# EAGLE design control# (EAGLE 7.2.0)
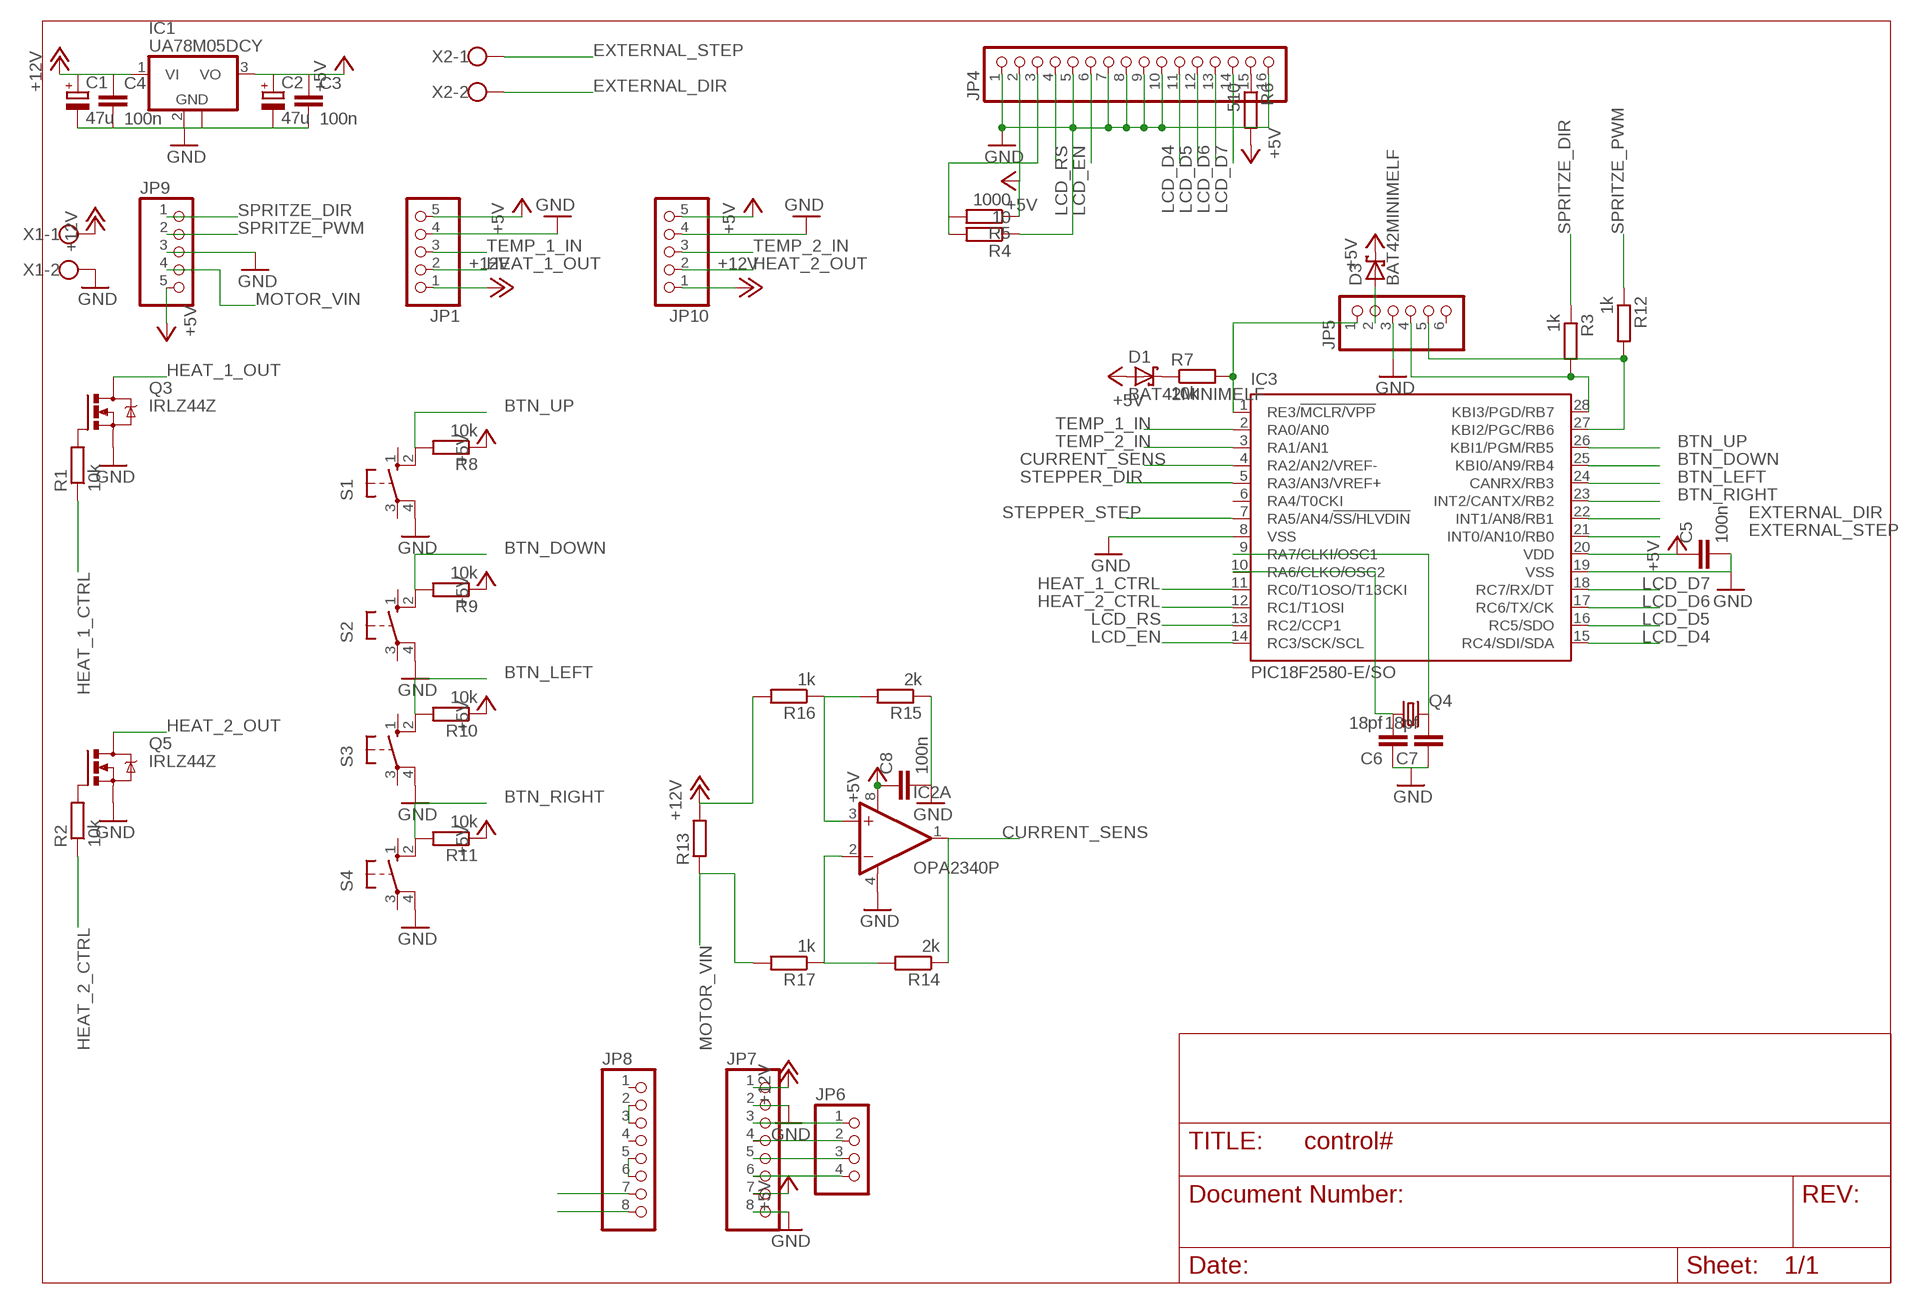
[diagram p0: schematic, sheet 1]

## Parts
C1  47u  CPOL-EU153CLV-0605  [153CLV-0605]
C2  47u  CPOL-EU153CLV-0605  [153CLV-0605]
C3  100n  C-EUC0603  [C0603]
C4  100n  C-EUC0603  [C0603]
C5  100n  C-EUC0603  [C0603]
C6  18pf  C-EUC0603  [C0603]
C7  18pf  C-EUC0603  [C0603]
C8  100n  C-EUC0603  [C0603]
D1  BAT42MINIMELF  [MINIMELF]
D3  BAT42MINIMELF  [MINIMELF]
IC1  UA78M05DCY  [SOT223]
IC2  OPA2340P  [DIL08]
IC3  PIC18F2580-E/SO  [SO28W]
JP1  PINHD-1X5_2.54  [1X05]
JP4  PINHD-1X16_2.54  [1X16]
JP5  PINHD-1X6_2.54  [1X06]
JP6  PINHD-1X4_2.54  [1X04]
JP7  PINHD-1X8_2.54  [1X08]
JP8  PINHD-1X8_2.54  [1X08]
JP9  PINHD-1X5_2.54  [1X05]
JP10  PINHD-1X5_2.54  [1X05]
Q3  IRLZ44Z  [TO220BH]
Q4  CRYSTALCTS406  [CTS406]
Q5  IRLZ44Z  [TO220BH]
R1  10k  R-EU_R0402  [R0402]
R2  10k  R-EU_R0402  [R0402]
R3  1k  R-EU_R0402  [R0402]
R4  10  R-EU_R0402  [R0402]
R5  1000  R-EU_R0402  [R0402]
R6  510  R-EU_R0402  [R0402]
R7  10k  R-EU_R0402  [R0402]
R8  10k  R-EU_R0402  [R0402]
R9  10k  R-EU_R0402  [R0402]
R10  10k  R-EU_R0402  [R0402]
R11  10k  R-EU_R0402  [R0402]
R12  1k  R-EU_R0402  [R0402]
R13  R-EU_R6332W  [R6332W]
R14  2k  R-EU_R0402  [R0402]
R15  2k  R-EU_R0402  [R0402]
R16  1k  R-EU_R0402  [R0402]
R17  1k  R-EU_R0402  [R0402]
S1  10-XX  [B3F-10XX]
S2  10-XX  [B3F-10XX]
S3  10-XX  [B3F-10XX]
S4  10-XX  [B3F-10XX]
X1  W237-102  [W237-102]
X2  W237-102  [W237-102]

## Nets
+5V: C2.+ C3.1 C5.1 C8.1 D1.A D3.C IC1.3(VO) IC2.8(A:V+) IC3.20(VDD) JP1.5 JP4.2 JP7.7 JP9.5 JP10.5 R5.1 R6.2 R8.1 R9.1 R10.1 R11.1
+12V: C1.+ C4.1 IC1.1(VI) JP1.1 JP7.1 JP10.1 R13.2 R16.2 X1.1
BTN_DOWN: IC3.25(KBI0/AN9/RB4) R9.2 S2.2(S1)
BTN_LEFT: IC3.24(CANRX/RB3) R10.2 S3.2(S1)
BTN_RIGHT: IC3.23(INT2/CANTX/RB2) R11.2 S4.2(S1)
BTN_UP: IC3.26(KBI1/PGM/RB5) R8.2 S1.2(S1)
CURRENT_SENS: IC2.1(A:OUT) IC3.4(RA2/AN2/VREF-) R14.1
EXTERNAL_DIR: IC3.22(INT1/AN8/RB1) X2.2
EXTERNAL_STEP: IC3.21(INT0/AN10/RB0) X2.1
GND: C1.- C2.- C3.2 C4.2 C5.2 C6.1 C7.1 C8.2 IC1.2(GND) IC1.4(GND) IC2.4(A:V-) IC3.8(VSS) IC3.19(VSS) JP1.4 JP4.1 JP4.5 JP4.7 JP4.8 JP4.9 JP4.10 JP4.16 JP5.3 JP7.2 JP7.8 JP9.3 JP10.4 Q3.S Q5.S R4.1 R15.1 S1.4(P1) S2.4(P1) S3.4(P1) S4.4(P1) X1.2
HEAT_1_CTRL: IC3.11(RC0/T1OSO/T13CKI) R1.1
HEAT_1_OUT: JP1.2 Q3.D
HEAT_2_CTRL: IC3.12(RC1/T1OSI) R2.1
HEAT_2_OUT: JP10.2 Q5.D
LCD_D4: IC3.15(RC4/SDI/SDA) JP4.11
LCD_D5: IC3.16(RC5/SDO) JP4.12
LCD_D6: IC3.17(RC6/TX/CK) JP4.13
LCD_D7: IC3.18(RC7/RX/DT) JP4.14
LCD_EN: IC3.14(RC3/SCK/SCL) JP4.6
LCD_RS: IC3.13(RC2/CCP1) JP4.4
MOTOR_VIN: JP9.4 R13.1 R17.2
N$1: Q3.G R1.2
N$2: Q5.G R2.2
N$3: JP6.1 JP7.3
N$4: IC3.27(KBI2/PGC/RB6) JP5.5 R12.2
N$5: IC3.28(KBI3/PGD/RB7) JP5.4 R3.2
N$6: IC3.1(RE3/!MCLR/VPP) JP5.1 R7.2
N$7: D1.C R7.1
N$8: D3.A JP5.2
N$9: JP4.3 R4.2 R5.2
N$10: JP6.2 JP7.4
N$11: JP6.3 JP7.5
N$12: JP6.4 JP7.6
N$13: JP8.2 JP8.3
N$14: JP8.5 JP8.6
N$16: C6.2 IC3.10(RA6/CLKO/OSC2) Q4.1
N$17: JP4.15 R6.1
N$18: C7.2 IC3.9(RA7/CLKI/OSC1) Q4.3
N$19: IC2.2(A:-IN) R14.2 R17.1
N$20: IC2.3(A:+IN) R15.2 R16.1
SPRITZE_DIR: JP9.1 R3.1
SPRITZE_PWM: JP9.2 R12.1
STEPPER_DIR: IC3.5(RA3/AN3/VREF+) JP8.8
STEPPER_STEP: IC3.7(RA5/AN4/!SS/HLVDIN) JP8.7
TEMP_1_IN: IC3.2(RA0/AN0) JP1.3
TEMP_2_IN: IC3.3(RA1/AN1) JP10.3
Unconnected: IC2.5(B:+IN) IC2.6(B:-IN) IC2.7(B:OUT) IC3.6(RA4/T0CKI) JP5.6 JP8.1 JP8.4 S1.1(S) S1.3(P) S2.1(S) S2.3(P) S3.1(S) S3.3(P) S4.1(S) S4.3(P)

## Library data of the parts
C1 C2 = rcl:CPOL-EU: POLARIZED CAPACITOR, European symbol
C3-C8 = rcl:C-EU: CAPACITOR, European symbol
D1 D3 = fab-pic:BAT42: DIODE
IC1 = linear:UA78M*: POSITIVE-VOLTAGE REGULATORS Source: http://focus.ti.com/lit/ds/symlink/ua78m33.pdf
IC2 = burr-brown:OPA2340: Single-Supply, Rail-to-Rail Operational Amplifiers MicroAmplifier(TM) Series; Product Folder:OPA2340; MF: TEXAS INSTRUMENTS; MPN: OPA2340PA; OC_FARNELL: 1129252; OC_NEWARK: 62K3460
IC3 = microchip:PIC18F2*80: 28-Pin Enhanced Flash Microcontrollers with ECAN(TM) Technology 10-Bit A/D and nanoWatt Technology Source: http://www.microchip.com .. 39637a.pdf; MF: MICROCHIP; MPN: PIC18F2580-I/SO; OC_FARNELL: 9321284; OC_NEWARK: 71J7243
JP1 JP9 JP10 = pinhead:PINHD-1X5: PIN HEADER
JP4 = pinhead:PINHD-1X16: PIN HEADER
JP5 = pinhead:PINHD-1X6: PIN HEADER
JP6 = pinhead:PINHD-1X4: PIN HEADER
JP7 JP8 = pinhead:PINHD-1X8: PIN HEADER
Q3 Q5 = transistor-power:IRLZ44Z: N-Channel HEXFET® Power MOSFET Logic Level AUTOMOTIVE MOSFET Source: http://www.irf.com/product-info/datasheets/data/irlz44zpbf.pdf
Q4 = fab-pic:CRYSTAL: CRYSTAL; OC_FARNELL: unknown; OC_NEWARK: unknown
R1-R17 = rcl:R-EU_: RESISTOR, European symbol
S1-S4 = fab-pic:10-XX: OMRON SWITCH; MPN: B3F-1000; OC_FARNELL: 176432; OC_NEWARK: 36M3542
X1 X2 = con-wago-500:W237-102: WAGO SCREW CLAMP; MPN: 237-102; OC_FARNELL: unknown; OC_NEWARK: 70K9898

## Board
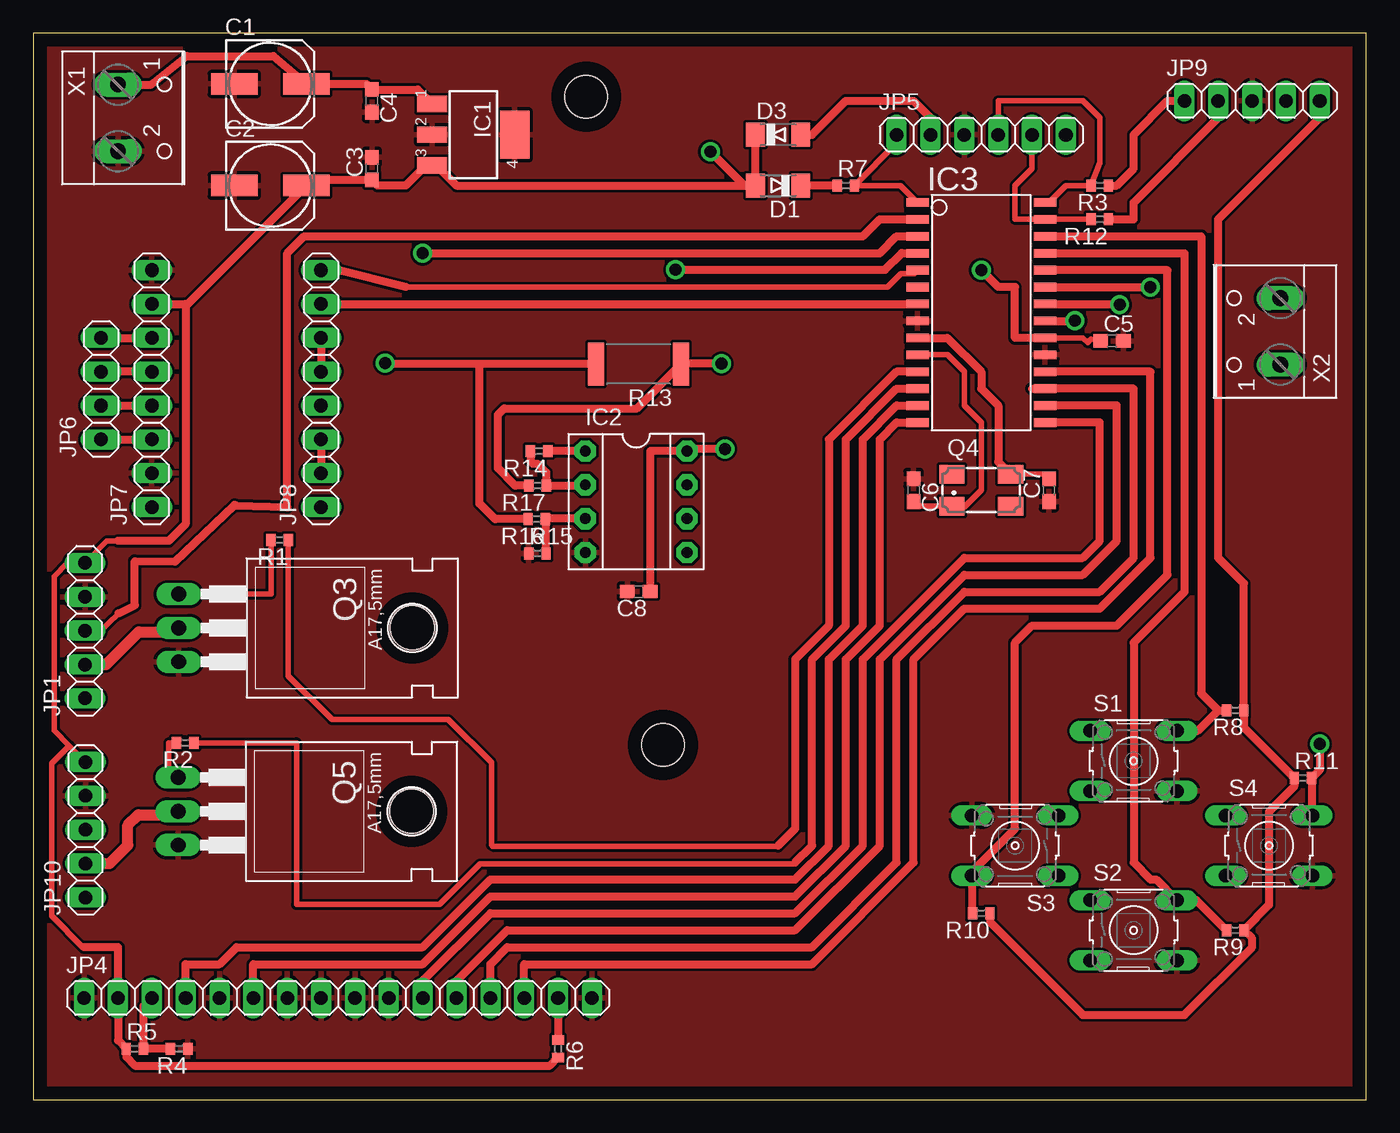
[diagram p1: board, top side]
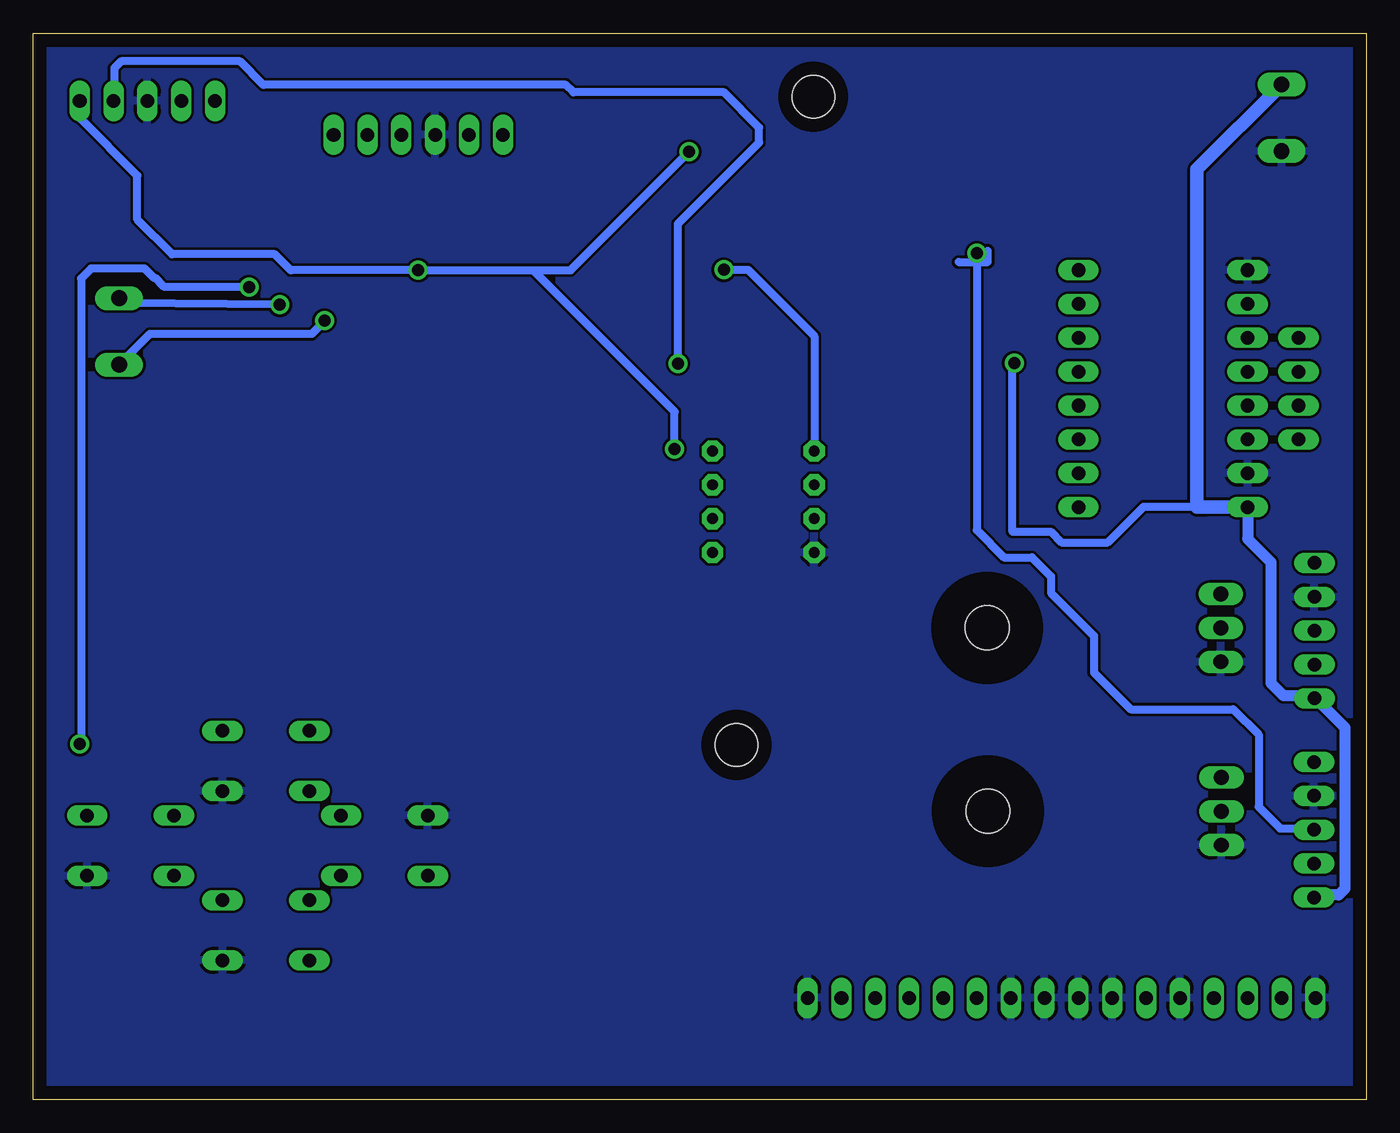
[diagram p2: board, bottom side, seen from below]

Size 100 x 80 mm. Coordinates in mm from the lower left corner, seen from the top.
Outline: 0,0 100,0 100,80 0,80 0,0
Copper layers (1*16): Top 0.035mm / dielectric 1.5mm / Bottom 0.035mm
Design rules "default": minimum track width 10mil, minimum drill 24mil, track to track 8mil, track to pad 8mil, pad to pad 8mil, via to via 8mil, smd to smd 8mil, copper to edge 40mil, drill to drill 8mil, minimum pad ring 10mil, minimum via ring 8mil, stop-mask expansion 4mil, vias tented up to drill 0mil, thermal gap 10mil
Holes 3.2 mm at 41.48,75.25 47.24,26.6

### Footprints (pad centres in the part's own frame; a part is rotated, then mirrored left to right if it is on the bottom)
153CLV-0605 = smd 3.5 x 1.6: + 2.7,0; - -2.7,0
C0603 = smd 1.1 x 1: 1 -0.85,0; 2 0.85,0
MINIMELF = smd 1.4 x 1.8: A 1.7,0; C -1.7,0
SOT223 = smd 1.219 x 2.235: 1 -2.311,-3.099; 2 0,-3.099; 3 2.311,-3.099 | smd 3.6 x 2.2: 4 0,3.099
DIL08 = drill 0.813 pad 1.6 octagon: 1 -3.81,-3.81; 2 -1.27,-3.81; 3 1.27,-3.81; 4 3.81,-3.81; 5 3.81,3.81; 6 1.27,3.81; 7 -1.27,3.81; 8 -3.81,3.81
SO28W = smd 0.65 x 1.7: 1 -7.62,-4.78; 2 -6.35,-4.78; 3 -5.08,-4.78; 4 -3.81,-4.78; 5 -2.54,-4.78; 6 -1.27,-4.78; 7 0,-4.78; 8 1.27,-4.78; 9 2.54,-4.78; 10 3.81,-4.78; 11 5.08,-4.78; 12 6.35,-4.78; 13 7.62,-4.78; 14 8.89,-4.78; 15 8.89,4.78; 16 7.62,4.78; 17 6.35,4.78; 18 5.08,4.78; 19 3.81,4.78; 20 2.54,4.78; 21 1.27,4.78; 22 0,4.78; 23 -1.27,4.78; 24 -2.54,4.78; 25 -3.81,4.78; 26 -5.08,4.78; 27 -6.35,4.78; 28 -7.62,4.78
1X05 = drill 1.016 long: 1 -5.08,0; 2 -2.54,0; 3 0,0; 4 2.54,0; 5 5.08,0
1X16 = drill 1.016 long: 1 -19.05,0; 2 -16.51,0; 3 -13.97,0; 4 -11.43,0; 5 -8.89,0; 6 -6.35,0; 7 -3.81,0; 8 -1.27,0; 9 1.27,0; 10 3.81,0; 11 6.35,0; 12 8.89,0; 13 11.43,0; 14 13.97,0; 15 16.51,0; 16 19.05,0
1X06 = drill 1.016 long: 1 -6.35,0; 2 -3.81,0; 3 -1.27,0; 4 1.27,0; 5 3.81,0; 6 6.35,0
1X04 = drill 1.016 long: 1 -3.81,0; 2 -1.27,0; 3 1.27,0; 4 3.81,0
1X08 = drill 1.016 long: 1 -8.89,0; 2 -6.35,0; 3 -3.81,0; 4 -1.27,0; 5 1.27,0; 6 3.81,0; 7 6.35,0; 8 8.89,0
TO220BH = drill 1.118 long: D 0,-6.35; G -2.54,-6.35; S 2.54,-6.35 | hole 3.302: 0,11.176
CTS406 = smd 1.9 x 1.4: 1 -2.2,-1.2; 2 2.2,-1.2; 3 2.2,1.2; 4 -2.2,1.2
R0402 = smd 0.7 x 0.9: 1 -0.65,0; 2 0.65,0
R6332W = smd 1.2 x 3.2: 1 -3.196,0; 2 3.196,0
B3F-10XX = drill 1.016 long: 1 -3.251,2.261; 2 3.251,2.261; 3 -3.251,-2.261; 4 3.251,-2.261
W237-102 = drill 1.194 long: 1 -2.5,-1.27; 2 2.5,-1.27

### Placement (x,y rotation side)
C1  17.78,76.2 0 top
C2  17.78,68.58 0 top
C3  25.4,69.85 90 top
C4  25.4,74.93 270 top
C5  80.94,56.92 0 top
C6  66.04,45.72 270 top
C7  76.2,45.72 90 top
C8  45.42,38.12 180 top
D1  55.88,68.58 180 top
D3  55.88,72.39 0 top
IC1  33.02,72.39 270 top
IC2  45.23,44.85 270 top
IC3  71.12,59.69 270 top
JP1  3.88,35.18 90 top
JP4  22.86,7.62 0 top
JP5  71.12,72.39 0 top
JP6  5.08,53.34 90 top
JP7  8.89,53.34 90 top
JP8  21.59,53.34 90 top
JP9  91.44,74.93 0 top
JP10  3.91,20.24 90 top
Q3  17.26,35.39 270 top
Q4  71.12,45.72 0 top
Q5  17.21,21.63 270 top
R1  18.48,41.99 180 top
R2  11.39,26.76 180 top
R3  80.01,68.58 180 top
R4  10.94,3.81 180 top
R5  7.62,3.81 0 top
R6  39.37,3.81 270 top
R7  60.96,68.58 0 top
R8  90.17,29.21 180 top
R9  90.17,12.7 180 top
R10  71.12,13.97 180 top
R11  95.25,24.13 0 top
R12  80.01,66.04 180 top
R13  45.41,55.18 180 top
R14  37.95,48.64 180 top
R15  37.82,40.99 0 top
R16  37.77,43.54 180 top
R17  37.83,46.06 180 top
S1  82.55,25.4 0 top
S2  82.55,12.7 0 top
S3  73.66,19.05 180 top
S4  92.71,19.05 0 top
X1  7.62,73.66 270 top
X2  92.3,57.63 90 top

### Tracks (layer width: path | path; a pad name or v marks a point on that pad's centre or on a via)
+5V  (via drill 0.9 pad 1.42)
  Top 0.406: IC3.20 78.74,57.15 79.11,56.78 79.36,57.06 C5.1 | 6.35,41.91 5.52,41.91 JP1.5 2.56,40.26 1.56,39.26 1.56,27.68 2.7,26.54 | 2.7,26.54 JP10.5 | 3.81,11.43 3.72,11.43 1.37,13.77 1.37,25.21 2.7,26.54
  Top 0.61: IC3.20 73.66,57.15 73.66,60.96 72.39,60.96 v71.12,62.23 | R10.1 71.77,13.32 78.74,6.35 86.36,6.35 91.44,11.43 91.44,12.08 R9.1 92.71,14.59 92.71,21.59 94.6,23.48 R11.1 90.82,27.91 R8.1 90.82,38.72 88.9,40.64 88.9,66.04 96.52,73.66 JP9.5 | 53.34,68.58 31.75,68.58 30.25,70.08 IC1.3 29.44,70.08 27.94,68.58 25.82,68.58 C3.1 20.9,69 C2.+ 11.59,59.69 11.43,59.69 | 53.34,68.58 D1.A D3.C | v50.8,71.12 53.34,68.58 | JP7.7 11.43,59.69 | 11.43,59.69 11.43,43.18 10.16,41.91 6.35,41.91 | 3.81,11.43 6.35,11.43 JP4.2 6.35,4.43 R5.1 6.97,3.19 7.62,2.54 38.75,2.54 R6.2 | C8.1 46.27,48.63 46.31,48.66 IC2.8 49.19,48.81 v51.89,48.81 | C8.1
  Bottom 0.61: 62.51,62.23 v71.12,62.23 80.69,62.23 81.89,63.43 89.58,63.43 92.19,66.04 92.19,69.33 96.45,73.59 96.45,74.86 JP9.5 | 62.51,62.23 59.69,62.23 v50.8,71.12 | v51.89,48.81 51.89,51.61 62.51,62.23
+12V  (via drill 0.9 pad 1.42)
  Top 0.61: X1.1 8.85,76.16 11.52,78.29 18.03,78.29 C1.+ 24.98,76.2 C4.1 28.84,75.78 IC1.1 | R13.2 33.4,55.18 | 33.4,55.18 26.47,55.18 v26.4,55.25 | R16.2 34.64,43.54 33.47,44.72 33.47,55.11 33.4,55.18
  Bottom 0.61: v26.4,55.25 26.54,55.12 26.54,42.6 23.67,42.6 22.87,41.8 19.39,41.8 16.7,44.49 12.14,44.49 12.11,44.45
  Bottom 0.813: JP7.1 8.89,42.07 7.14,40.31 7.14,31.25 6.21,30.32 4.09,30.32 JP1.1 3.79,30.1 1.59,27.9 1.59,15.82 2.06,15.34 3.73,15.34 JP10.1
  Bottom 1.016: JP7.1 12.11,44.45 12.7,44.45 12.7,69.81 X1.1
BTN_DOWN
  Top 0.61: IC3.25 86.36,63.5 86.36,38.1 82.55,34.29 82.55,17.78 83.82,16.51 84.25,16.51 S2.2 87.26,14.96 R9.2
BTN_LEFT
  Top 0.61: IC3.24 85.09,62.23 85.09,39.37 81.28,35.56 74.93,35.56 73.66,34.29 73.66,20.32 70.41,17.07 S3.2 70.41,14.03 R10.2
BTN_RIGHT  (via drill 0.9 pad 1.42)
  Top 0.61: IC3.23 v83.82,60.96 | v96.52,26.67 96.52,24.75 R11.2 95.9,21.37 S4.2
  Bottom 0.61: v83.82,60.96 90.17,60.96 90.87,61.66 90.95,61.66 91.65,62.36 95.66,62.36 96.42,61.6 96.42,27 96.46,26.96 96.46,26.73 v96.52,26.67
BTN_UP
  Top 0.61: IC3.26 87.63,64.77 87.63,30.48 88.9,29.21 | 88.9,29.21 R8.2 | S1.2 87.35,27.66 88.9,29.21
CURRENT_SENS  (via drill 0.9 pad 1.42)
  Top 0.61: v48.19,62.26 63.9,62.26 65.15,63.51 66.33,63.51 IC3.4 | IC2.1 38.62,48.66 R14.1
  Bottom 0.61: v48.19,62.26 46.37,62.26 41.4,57.29 41.4,48.68 IC2.1
EXTERNAL_DIR  (via drill 0.9 pad 1.42)
  Top 0.61: IC3.22 81.09,59.69 v81.5,59.63
  Bottom 0.61: v81.5,59.63 93.3,59.74 X2.2
EXTERNAL_STEP  (via drill 0.9 pad 1.42)
  Top 0.61: IC3.21 78.14,58.42 v78.16,58.44
  Bottom 0.61: v78.16,58.44 78.16,58.39 79.12,57.43 91.26,57.43 X2.1
GND
  pour Top: -1.27,81.28 101.6,81.28 101.6,-3.81 -1.27,-3.81
  pour Bottom: -7.62,83.82 106.68,83.82 106.68,-8.89 -7.62,-8.89
HEAT_1_CTRL
  Top 0.406: R1.1 19.13,31.79 22.41,28.52 31.14,28.52 34.37,25.29 34.37,19.11 34.46,19.01 55.84,19.01 56.12,19.29
  Top 0.61: IC3.11 64.77,54.61 59.69,49.53 59.69,35.56 57.15,33.02 57.15,20.32 56.12,19.29 55.88,19.05
HEAT_1_OUT
  Top 0.813: JP1.2 5.46,32.64 7.92,35.1 10.62,35.1 Q3.D
HEAT_2_CTRL
  Top 0.406: R2.1 19.75,26.77 19.75,14.64 30.47,14.64 33.52,17.68 57.05,17.68 57.15,17.78
  Top 0.61: 57.15,17.78 58.42,19.05 58.42,33.02 60.96,35.56 60.96,49.53 64.77,53.34 IC3.12
HEAT_2_OUT
  Top 0.813: JP10.2 5.72,17.7 7.09,19.08 7.09,20.59 7.87,21.37 10.6,21.37 Q5.D
LCD_D4
  Top 0.61: JP4.11 29.21,8.89 34.29,13.97 57.15,13.97 62.23,19.05 62.23,33.02 69.85,40.64 78.74,40.64 80.01,41.91 80.01,50.8 IC3.15
LCD_D5
  Top 0.61: JP4.12 31.75,8.89 35.56,12.7 57.15,12.7 63.5,19.05 63.5,33.02 69.85,39.37 78.74,39.37 81.28,41.91 81.28,52.07 IC3.16
LCD_D6
  Top 0.61: JP4.13 34.29,10.16 35.56,11.43 58.42,11.43 64.77,17.78 64.77,33.02 69.85,38.1 80.01,38.1 82.55,40.64 82.55,53.34 IC3.17 74.93,53.34
LCD_D7
  Top 0.61: JP4.14 36.83,10.16 58.42,10.16 66.04,17.78 66.04,33.02 69.85,36.83 80.01,36.83 83.82,40.64 83.82,54.61 IC3.18
LCD_EN
  Top 0.61: JP4.6 16.51,10.16 29.21,10.16 34.29,15.24 57.15,15.24 60.96,19.05 60.96,33.02 63.5,35.56 63.5,49.53 64.77,50.8 IC3.14
LCD_RS
  Top 0.61: JP4.4 11.43,10.16 13.97,10.16 15.24,11.43 29.21,11.43 34.29,16.51 57.15,16.51 59.69,19.05 59.69,33.02 62.23,35.56 62.23,49.53 64.77,52.07 IC3.13
MOTOR_VIN  (via drill 0.9 pad 1.42)
  Top 0.61: R17.2 36.16,46.06 34.85,47.37 34.85,51.38 35.33,51.86 45.28,51.86 R13.1 48.64,55.22 v51.63,55.22
  Bottom 0.61: v51.63,55.22 51.63,65.71 45.54,71.81 45.54,72.94 48.18,75.58 59.49,75.58 60.05,76.14 82.74,76.14 84.5,77.9 93.42,77.9 93.92,77.4 93.92,74.99 JP9.4
N$1
  Top 0.406: Q3.G 17.83,37.93 R1.2
N$2
  Top 0.406: R2.2 10.16,26.77 10.16,24.07 10.86,24.07 Q5.G
N$3
  Top 0.61: JP6.1 JP7.3
N$4
  Top 0.406: JP5.5 74.93,69.85 73.66,68.58 73.66,66.04 IC3.27 R12.2
N$5
  Top 0.406: JP5.4 72.39,74.93 78.74,74.93 80.01,73.66 80.02,70.28 R3.2 77.47,68.58 76.2,67.31 IC3.28
N$6
  Top 0.406: JP5.1 64.77,71.74 R7.2 65.07,68.58 IC3.1
N$7
  Top 0.61: R7.1 D1.C
N$8
  Top 0.61: D3.A 58.42,72.39 60.96,74.93 66.04,74.93 67.31,73.66 JP5.2
N$9
  Top 0.61: R4.2 R5.2 8.27,7 JP4.3
N$10
  Top 0.61: JP6.2 JP7.4
N$11
  Top 0.61: JP7.5 JP6.3
N$12
  Top 0.61: JP6.4 JP7.6
N$13
  Top 0.61: JP8.3 JP8.2
N$14
  Top 0.61: JP8.6 JP8.5
N$15
  Bottom 0.61: 30.58,62.83 28.4,62.83 28.4,63.69
N$16
  Top 0.406: IC3.10 68.58,55.88 69.85,54.61 69.85,52.07 71.12,50.8 71.12,45.72 69.85,44.45 68.99,44.45 Q4.1 66.39,44.52 C6.2
N$17
  Top 0.61: JP4.15 R6.1
N$18
  Top 0.406: 72.82,47.42 Q4.3 75.85,46.92 C7.2
  Top 0.61: IC3.9 68.58,57.15 71.12,54.61 71.12,53.34 72.39,52.07 72.39,47.85 72.82,47.42
N$19
  Top 0.61: R14.2 37.3,47.89 37.47,47.72 37.82,47.72 38.47,47.06 R17.1 41.36,46.06 IC2.2
N$20
  Top 0.61: IC2.3 38.46,43.58 R16.1 38.42,41.04 R15.2
SPRITZE_DIR
  Top 0.61: R3.1 81.28,68.58 82.55,69.85 82.55,72.39 85.09,74.93 JP9.1
SPRITZE_PWM
  Top 0.61: R12.1 82.55,66.04 82.55,67.31 88.9,73.66 JP9.2
STEPPER_DIR
  Top 0.406: 27.94,60.96 64.08,60.96 65.1,61.98 66.09,61.98 IC3.5
  Top 0.61: 27.94,60.96 22.86,62.23 JP8.8
STEPPER_STEP
  Top 0.61: JP8.7 IC3.7
TEMP_1_IN
  Top 0.406: 6.4,36.49 4.81,34.98 JP1.3
  Top 0.61: 6.4,36.49 7.62,37.07 7.62,40.4 10.64,40.36 15.1,44.61 15.18,44.57 19.05,44.45 19.05,63.5 20.32,64.77 62.23,64.77 63.5,66.04 IC3.2
TEMP_2_IN  (via drill 0.9 pad 1.42)
  Top 0.61: v29.21,63.5 63.5,63.5 64.77,64.77 IC3.3
  Bottom 0.61: v29.21,63.5 29.21,42.73 27.16,40.68 25.07,40.68 23.65,39.26 23.65,38.02 20.42,34.79 20.42,32.03 17.67,29.28 9.97,29.28 8.07,27.38 8.07,21.96 6.46,20.34 4.01,20.34 JP10.3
